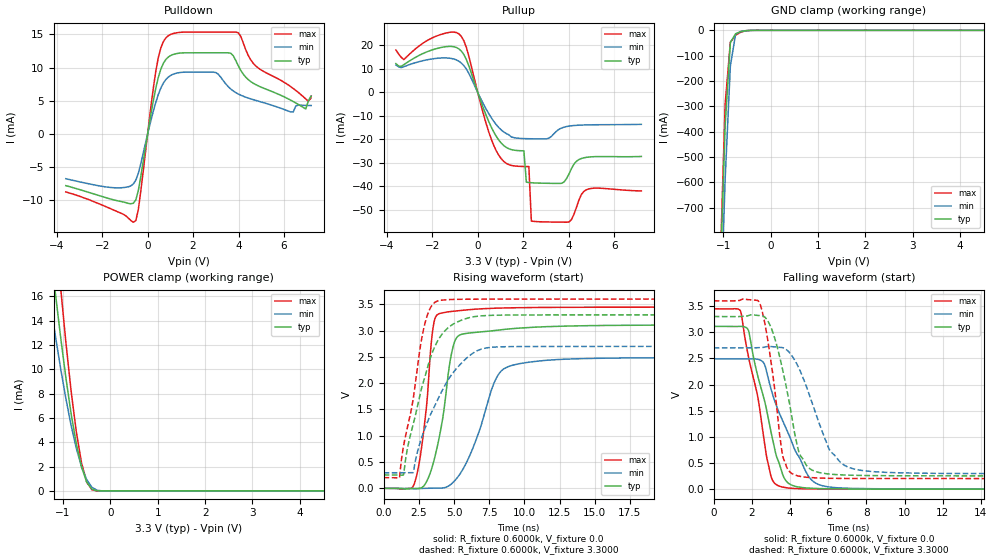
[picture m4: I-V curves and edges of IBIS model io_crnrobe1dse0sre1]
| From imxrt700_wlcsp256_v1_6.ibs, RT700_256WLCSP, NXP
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[Model] io_crnrobe1dse0sre1
|   Model io_crnrobe1dse0sre1
| This model was characterised for following simulation conditions:
| External (pad) voltage:
|   - Typ: 3.3V,   - Min: 2.7V,   - Max: 3.6V
| Library cells for typ/min/max conditions are connected as defined below:
|  PAD_IO - External Pad
|  ipp_do - Core Input
|  ipp_obe - Output Buffer Enable
|  ASRCN3V3[3] - NC
|  ASRCN3V3[4] - NC
|  ASRCP3V3[4] - NC
|  REFAPBIAS3V3 - gnde
|  REFBAMPL3V3 - vdd1v8
|  REFCAMPH3V3 - vdd1v8
|  REFDNBIAS3V3 - vdd1v8
|  REFH3V3 - REFH3V3
|  REFL3V3 - REFL3V3
|  gnde - gnde
|  ipp_dse - gnde
|  ipp_ina235_3v - NC
|  ipp_ina40_3v - NC
|  ipp_ina_mux - NC
|  ipp_ind - NC
|  ipp_ind_1p8v - NC
|  ipp_ind_3v - NC
|  ipp_sre - vdd
|  vdd - vdd
|  vdd1v8 - vdd1v8
|  vdda - vdde3v3
|  vdde3v3 - vdde3v3
| All other pins connected to ground
Model_type I/O
Polarity   Non-Inverting
Enable   Active-High
Vinl =   0.9900V
Vinh =   2.3100V
Vmeas =  1.6500V
Cref =   15.0000pF
Rref =   0.6000k
Vref =   0.0V
C_comp   4.0038pF   3.8208pF   4.1229pF
|C_comp_pullup   0.5150pF   0.5957pF   0.4948pF
|C_comp_pulldown   2.0815pF   2.1738pF   1.8626pF
[Model Spec]
| variable   typ   min   max
Vinh   2.3100V   NA   NA
Vinl   0.9900V   NA   NA
Vref   0.0V   0.0V   0.0V
Cref   15.0000pF   15.0000pF   15.0000pF
Rref   0.6000k   0.6000k   0.6000k
[Receiver Thresholds]
Vcross_high  =   0.0V
Vcross_low  =   0.0V
Vdiff_ac  =   0.0V
Vdiff_dc  =   0.0V
Tdiffslew_ac  =   0.0S
[Temperature Range]   25.0000   0.1250k   -40.0000
[Voltage Range]   3.3000V   2.7000V   3.6000V
[Pullup Reference]   3.3000V   2.7000V   3.6000V
[Pulldown Reference]   0.0V   0.0V   0.0V
[POWER Clamp Reference]   3.3000V   2.7000V   3.6000V
[GND Clamp Reference]   0.0V   0.0V   0.0V
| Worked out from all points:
|   slope of the pulldown table from 0 to 0.495 V, typ, clamps not added: 56.2 ohm
|   slope of the pullup table from 0 to 0.495 V, typ, clamps not added: 39.2 ohm
|   GND clamp passes 1 mA (typ) near -0.49 V on its own axis
|   POWER clamp passes 1 mA (typ) near -0.52 V on its own axis
|   rising waveform, R_fixture 0.6000k, V_fixture 0.0: 20-80 % time 1.1ns typ, 1.93ns min, 731ps max; typ from 0 V to 3.11 V
|   rising waveform, R_fixture 0.6000k, V_fixture 3.3000: 20-80 % time 1.85ns typ, 2.51ns min, 1.29ns max; typ from 0.254 V to 3.3 V
|   falling waveform, R_fixture 0.6000k, V_fixture 0.0: 20-80 % time 1.19ns typ, 1.68ns min, 1.04ns max; typ from 3.11 V to 0 V
|   falling waveform, R_fixture 0.6000k, V_fixture 3.3000: 20-80 % time 1.01ns typ, 1.46ns min, 713ps max; typ from 3.3 V to 0.254 V
[Pulldown]
|Voltage   I(typ)   I(min)   I(max)
-3.6V     -7.78mA    -6.73mA    -8.72mA
-1.4V     -9.994mA   -8.102mA   -11.59mA
-520mV    -9.932mA   -6.949mA   -13.06mA
470mV     8.52mA     5.95mA     11.49mA
1.02V     11.84mA    8.844mA    15.02mA
3V        12.25mA    9.26mA     15.36mA
3.66V     12.17mA    6.782mA    15.36mA
3.99V     10.29mA    6.033mA    15.27mA
4.76V     7.445mA    5.07mA     10.26mA
6.3V      5.098mA    3.32mA     7.14mA
6.96V     3.779mA    4.318mA    5.29mA
7.2V      5.692mA    4.298mA    5.697mA
[Pullup]
|Voltage   I(typ)   I(min)   I(max)
-3.6V     12.26mA    11.64mA    18.04mA
-3.25V    11.82mA    10.96mA    13.98mA
-1.82V    18.63mA    14.49mA    23.96mA
-720mV    17.58mA    12.47mA    23.82mA
820mV     -18.75mA   -13.76mA   -24.91mA
2.03V     -24.84mA   -19.63mA   -31.51mA
2.14V     -38.17mA   -19.67mA   -31.53mA
2.25V     -38.32mA   -19.69mA   -31.54mA
2.36V     -38.42mA   -19.71mA   -54.75mA
4.01V     -34.78mA   -14.34mA   -55.12mA
4.89V     -27.48mA   -13.8mA    -41.02mA
7.2V      -27.24mA   -13.57mA   -41.9mA
[GND_clamp]
|Voltage   I(typ)   I(min)   I(max)
-3.6V     -19.67A    -19.55A    -20.65A
-1.07V    -1.013A    -1.224A    -956.3mA
-960mV    -377.1mA   -587.4mA   -291.7mA
-850mV    -48.2mA    -140.8mA   -46.94mA
-740mV    -13.57mA   -15.62mA   -19.22mA
-630mV    -5.136mA   -4.37mA    -7.235mA
-520mV    -1.276mA   -1.53mA    -1.554mA
-300mV    -4.356uA   -32.48uA   -995.7nA
7.2V      0A         0A         0A
[POWER_clamp]
|Voltage   I(typ)   I(min)   I(max)
-3.6V     102.7mA    81.65mA    131.1mA
-1.38V    23.95mA    18.52mA    31.78mA
-1.27V    20.01mA    15.56mA    26.56mA
-1.16V    16.22mA    12.73mA    21.52mA
-1.05V    12.64mA    10.07mA    16.71mA
-830mV    6.384mA    5.406mA    8.254mA
-720mV    3.9mA      3.518mA    4.888mA
-610mV    1.982mA    2.008mA    2.327mA
-500mV    727.2uA    927.8uA    733.5uA
-390mV    144.5uA    302.5uA    95.96uA
-170mV    198.4nA    4.047uA    20.3nA
7.2V      0A         0A         0A
[Ramp]
| variable   typ   min   max
dV/dt_r  1.8668/1.1025n   1.4947/1.9292n   2.0685/0.7310n
dV/dt_f  1.8274/1.0132n   1.4426/1.4553n   2.0384/0.7128n
R_load = 0.6000k
[Rising Waveform]
R_fixture= 0.6000k
V_fixture= 0.0
V_fixture_min= 0.0
V_fixture_max= 0.0
|time   V(typ)   V(min)   V(max)
0s        139.9nV    3.471uV    132.7nV
2.22ns    -5.09mV    -8.805mV   119.8mV
2.868ns   49.75mV    -952.4uV   1.134V
3.53ns    482.9mV    320uV      3.085V
4.168ns   1.284V     6.194mV    3.337V
4.75ns    2.465V     68.72mV    3.362V
5.23ns    2.881V     200.9mV    3.375V
8.092ns   3.009V     2.137V     3.427V
9.866ns   3.051V     2.381V     3.437V
60ns      3.111V     2.491V     3.448V
[Rising Waveform]
R_fixture= 0.6000k
V_fixture= 3.3000
V_fixture_min= 2.7000
V_fixture_max= 3.6000
|time   V(typ)   V(min)   V(max)
0s        254.3mV    295.6mV    202.7mV
1.126ns   253.4mV    295.5mV    206.6mV
1.42ns    265.1mV    295mV      814.7mV
2.095ns   1.212V     298.8mV    1.69V
2.866ns   2.06V      1.09V      3.062V
3.363ns   2.515V     1.423V     3.453V
3.912ns   2.839V     1.728V     3.571V
5.893ns   3.232V     2.476V     3.597V
7.707ns   3.291V     2.684V     3.599V
60ns      3.3V       2.7V       3.6V
[Falling Waveform]
R_fixture= 0.6000k
V_fixture= 0.0
V_fixture_min= 0.0
V_fixture_max= 0.0
|time   V(typ)   V(min)   V(max)
0s        3.111V     2.491V     3.447V
1.386ns   3.112V     2.491V     3.415V
1.809ns   3.041V     2.489V     2.545V
2.308ns   2.16V      2.483V     1.761V
2.599ns   1.774V     2.422V     1.033V
3ns       1.091V     1.913V     244.6mV
3.803ns   151.1mV    1.151V     26.98mV
5.082ns   17.58mV    192.5mV    3.931mV
6.526ns   5.133mV    25.2mV     706.4uV
60ns      2.332uV    9.792uV    1.996uV
[Falling Waveform]
R_fixture= 0.6000k
V_fixture= 3.3000
V_fixture_min= 2.7000
V_fixture_max= 3.6000
|time   V(typ)   V(min)   V(max)
0s        3.3V       2.7V       3.6V
2.382ns   3.318V     2.705V     3.571V
2.909ns   3.163V     2.728V     2.661V
3.616ns   2.269V     2.704V     633.1mV
3.954ns   1.666V     2.615V     341.5mV
4.586ns   617.3mV    2.211V     240.1mV
6.083ns   287.7mV    742.4mV    207.5mV
6.906ns   269.8mV    444.7mV    204.4mV
8.127ns   260.2mV    342mV      203.1mV
60ns      254.3mV    295.6mV    202.7mV
